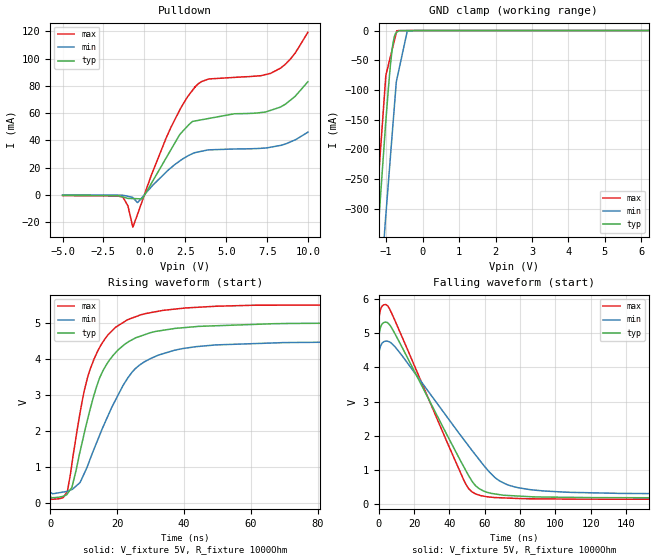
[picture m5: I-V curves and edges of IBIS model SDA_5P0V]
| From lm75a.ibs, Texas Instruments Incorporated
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|   Model SDA_5P0V
[Model]   SDA_5P0V
Model_type   I/O_open_drain
Polarity   Non-Inverting
Enable   Active-Low
Vinl = 1.5
Vinh = 3.5
Vmeas = 2.5
Vref = 5
Cref = 15pF
Rref = 1000
|   typ   min   max
|   (nom PVT)   (fast PVT)   (slow PVT)
C_comp   0.539p   0.494p   0.593p
|C_comp (ON state)   0.539p   0.494p   0.593p
|C_comp (OFF state)   0.638p   0.626p   0.666p
| Where   nom PVT is  Nominal Process, 5.0V, 27C
|   Fast PVT is Strong Process, 4.5V, -40C
|   Slow PVT is Weak Process, 5.5V, 150C
[Model spec]
|subparameter
Vinl   1.5   1.35   1.65
Vinh   3.5   3.15   3.85
[Voltage Range]   5   4.5   5.5
[Temperature Range]   27   150   -40
[Pullup Reference]   5   4.5   5.5
[Pulldown Reference]   0   0   0
[Power Clamp Reference]   5   4.5   5.5
[GND Clamp Reference]   0   0   0
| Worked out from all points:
|   slope of the pulldown table from 0 to 0.75 V, typ, clamps not added: 48.3 ohm
|   GND clamp passes 1 mA (typ) near -0.66 V on its own axis
|   falling waveform, V_fixture 5V, R_fixture 1000Ohm: 20-80 % time 28.9ns typ, 36.5ns min, 26.7ns max; typ from 5 V to 0.191 V
|   rising waveform, V_fixture 5V, R_fixture 1000Ohm: 20-80 % time 10.1ns typ, 13.2ns min, 8.83ns max; typ from 0.19 V to 5 V
[Pulldown]
|   Voltage   I(typ)   I(min)   I(max)
-5V       -417.2uA   -165.8uA   -573.8uA
-1.307V   -1.659mA   -358.3uA   -1.763mA
-1.007V   -2.672mA   -1.137mA   -8.142mA
-707.1mV  -2.792mA   -2.056mA   -23.79mA
-123.7mV  -3.026mA   -1.769mA   -4.285mA
1.313V    26.74mA    16.45mA    41.29mA
2.119V    43.51mA    24.46mA    61.33mA
3.08V     54.18mA    30.93mA    78.98mA
3.917V    56.03mA    32.98mA    85.07mA
7.713V    62.03mA    34.95mA    89.21mA
8.913V    69.45mA    38.81mA    99.62mA
9.985V    83.04mA    45.99mA    119.3mA
[GND Clamp]
|   Voltage   I(typ)   I(min)   I(max)
-5V       -3.855A    -3.902A    -3.838A
-1.314V   -419.6mA   -576.2mA   -339.8mA
-1.307V   -413.8mA   -570.4mA   -333.6mA
-1.021V   -163.5mA   -321.3mA   -87.07mA
-1.007V   -152.3mA   -310.7mA   -75.43mA
-901.3mV  -71.54mA   -227.9mA   -48.97mA
-845mV    -37.05mA   -183.9mA   -34.91mA
-770mV    -9.433mA   -125.2mA   -16.16mA
-720.7mV  -3.595mA   -86.58mA   -3.816mA
-707.1mV  -2.671mA   -82.72mA   -433.2uA
-420.7mV  -94.56uA   -1.179mA   -67.4uA
9.985V    0A         0A         0A
[Ramp]
R_load = 1000
|   typ   min   max
dV/dt_r   2.88588/1.00626e-08   2.51879/1.3162e-08   3.21044/8.82684e-09
dV/dt_f   2.88533/2.88717e-08   2.51711/3.64472e-08   3.21019/2.6675e-08
[Falling Waveform]
V_fixture = 5V
V_fixture_min = 4.5V
V_fixture_max = 5.5V
R_fixture = 1000Ohm
C_fixture = 0F
|   Time   V(typ)   V(min)   V(max)
0s        5V         4.5V       5.5V
1.322ns   5.22V      4.66V      5.742V
2.845ns   5.311V     4.752V     5.831V
6.071ns   5.247V     4.744V     5.714V
47.85ns   1.127V     1.914V     742.3mV
50.9ns    839.7mV    1.706V     460.7mV
55.15ns   532.9mV    1.421V     299.2mV
68.46ns   286mV      685.7mV    196mV
85.32ns   227.6mV    435.1mV    165.7mV
199.9ns   191.1mV    304.8mV    149.7mV
[Rising Waveform]
V_fixture = 5V
V_fixture_min = 4.5V
V_fixture_max = 5.5V
R_fixture = 1000Ohm
C_fixture = 0F
|   Time   V(typ)   V(min)   V(max)
0s        190.2mV    300.6mV    149.3mV
5.134ns   264.9mV    333.4mV    336.2mV
6.472ns   441.5mV    381.3mV    1.096V
10.13ns   1.928V     819.5mV    3.101V
14.31ns   3.356V     1.784V     4.24V
20.21ns   4.238V     2.985V     4.911V
27.04ns   4.628V     3.847V     5.214V
36.9ns    4.833V     4.229V     5.369V
49.48ns   4.912V     4.382V     5.452V
199.9ns   5V         4.499V     5.5V
